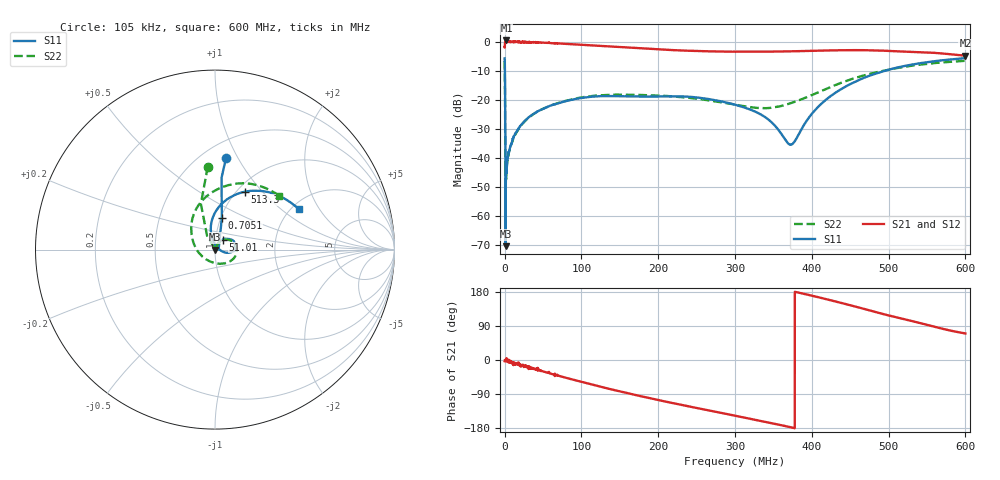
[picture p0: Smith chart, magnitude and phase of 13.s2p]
#  HZ  S  MA  R  50.00
! Rohde & Schwarz Vector Network Analyzer
! Rohde-Schwarz,ZNL6-2Port,1323001206101378,1.50.1.34-21.10.1.104
! Created: UTC 1/22/2024, 9:04:33 AM
! freq[Hz]  mag:S11  ang:S11  mag:S21  ang:S21  mag:S12  ang:S12  mag:S22  ang:S22
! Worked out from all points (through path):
!   5999 points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, 105 kHz to 600 MHz, reference 50 ohm
!   highest |S21| = 0.40 dB at 2.505 MHz (marker M1); lowest = -4.8 dB at 600 MHz (marker M2)
!   group delay of S21, straight-line fit = 1.29 ns
!   lowest |S11| = -70.5 dB at 1.505 MHz (marker M3), VSWR 1.00, Z = 50 + j0.0234 ohm
!   |S11| at or under -10 dB: 523.8 kHz to 495.6 MHz (495.1 MHz wide, 200 % of centre)
!   |S22| runs from -47.4 to -6.6 dB; largest |S21 - S12| = 0.25
!   S11 on the Smith chart (normalised r, x): 105 kHz: 0.64, +0.89; 705.1 kHz: 1.01, +0.37; 51.01 MHz: 1.08, +0.12; 513.3 MHz: 1.09, +0.81; 600 MHz: 2.19, +1.34
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105015.8  0.514 83.1  0.8062 -3.0  0.7644 -3.9  0.4645 95.0
705110.9  0.1806 77.8  0.9614 -0.0  0.947 -1.0  0.08834 119.8
1505238  0.0003001 51.2  1.004 -1.0  1.001 -0.8  0.007436 112.0
2505396  0.005391 76.5  1.047 4.9  0.9335 -8.1  0.005446 60.6
3505554  0.008734 62.2  0.9889 -2.6  1.006 -1.6  0.00845 61.1
4105649  0.009719 64.8  0.9958 -2.5  0.9978 -2.7  0.009381 61.8
9406489  0.01788 66.5  0.9853 -8.4  0.999 -4.2  0.01818 66.1
1.850793e7  0.03202 65.9  1.012 -7.0  0.9755 -15.5  0.03144 65.3
5.101308e7  0.0705 52.4  0.9581 -30.6  0.9553 -31.2  0.07051 50.1
1.001209e8  0.1071 31.1  0.8832 -57.7  0.8802 -58.5  0.1093 23.6
1.445279e8  0.1152 19.8  0.8139 -80.1  0.8084 -80.9  0.1219 4.5
2.001367e8  0.1135 4.4  0.7358 -105.6  0.734 -106.3  0.1181 -19.6
2.491444e8  0.1098 -3.1  0.69 -126.2  0.6897 -126.9  0.1044 -40.4
3.001525e8  0.08201 -12.0  0.6699 -147.0  0.6678 -147.7  0.0823 -73.0
3.405589e8  0.04871 -15.5  0.672 -163.6  0.669 -164.7  0.07153 -118.2
3.721639e8  0.01676 41.0  0.6807 -177.3  0.6793 -178.5  0.08665 -161.8
4.000683e8  0.05697 103.5  0.6942 169.7  0.6923 168.4  0.1201 166.0
4.410748e8  0.1597 96.6  0.711 149.2  0.7103 148.2  0.2018 129.9
5.000842e8  0.3283 69.2  0.6917 117.6  0.6869 116.9  0.3291 90.0
5.132863e8  0.3626 62.8  0.6789 111.0  0.6784 110.5  0.3551 81.8
5.485919e8  0.4403 46.4  0.6523 93.6  0.6555 92.1  0.4134 62.8
6e8  0.5184 25.6  0.5738 70.1  0.576 69.9  0.4677 39.9
